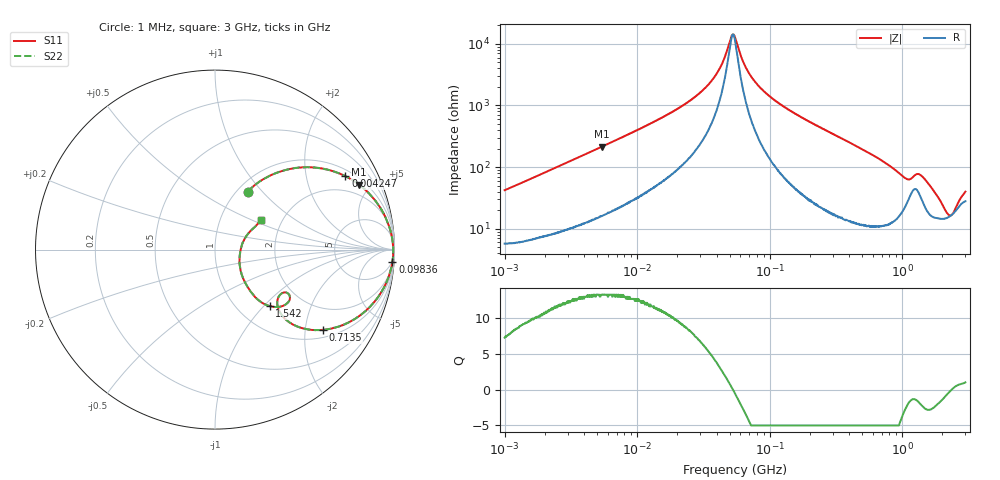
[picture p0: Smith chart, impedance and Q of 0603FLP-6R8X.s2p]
!s-Parameter Generated by FASTRON Sdn. Bhd.
!FASTRON P/N : 0603FLP-6R8X
!Keysight Technologies: E4991B_MY54100416_A.01.15
!Date: Tue Dec 02 13:07:44 2025
!Version  :Rev00  Tue Dec 02 13:07:44 2025
!Data & Calibration Information:
!Freq  S11  S21  S12  S22
!PortZ  Port1:50+j0  Port2:50+j0
!When reading reference impedance value at option line is always used.
! Remarks : This data is being provided solely for informational purposes.
# Hz S dB R 50
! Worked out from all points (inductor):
!   1601 points, 1 MHz to 3 GHz, reference 50 ohm
!   read as one part in series: L = 6.55 uH near 1.041 MHz
!   highest Q = 13.3 at 5.4 MHz (marker M1), where L = 6.29 uH
!   self-resonance near 52.62 MHz
!   S11 on the Smith chart (normalised r, x): 1 MHz: 1.11, +0.84; 4.247 MHz: 1.26, +3.38; 98.36 MHz: 4, -29; 713.5 MHz: 1.22, -2.50; 1.542 GHz: 1.39, -1.08; 3 GHz: 1.56, +0.57
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1000000  -8.60 60.6  -1.12 -21.6  -1.12 -21.6  -8.60 60.6
2128890  -4.06 46.2  -2.80 -38.6  -2.80 -38.6  -4.06 46.2
3804036  -1.86 32.0  -5.49 -53.6  -5.49 -53.6  -1.86 32.0
4246734  -1.58 29.4  -6.14 -56.2  -6.14 -56.2  -1.58 29.4
5399688  -1.10 24.2  -7.71 -61.5  -7.71 -61.5  -1.10 24.2
1.447069e7  -0.25 9.4  -15.70 -75.5  -15.70 -75.5  -0.25 9.4
3.371011e7  -0.08 2.7  -26.40 -77.2  -26.40 -77.2  -0.08 2.7
4.243531e7  -0.07 1.3  -32.50 -70.2  -32.50 -70.2  -0.07 1.3
5.15801e7  -0.06 0.1  -42.60 -19.8  -42.60 -19.8  -0.06 0.1
5.504702e7  -0.06 -0.2  -41.90 30.5  -41.90 30.5  -0.06 -0.2
6.929487e7  -0.06 -1.6  -30.80 75.2  -30.80 75.2  -0.06 -1.6
9.836149e7  -0.08 -3.9  -23.30 80.4  -23.30 80.4  -0.08 -3.9
2.083556e8  -0.24 -10.8  -14.60 76.2  -14.60 76.2  -0.24 -10.8
4.135554e8  -0.84 -22.0  -8.53 65.0  -8.53 65.0  -0.84 -22.0
7.135306e8  -2.50 -36.6  -4.46 48.3  -4.46 48.3  -2.50 -36.6
7.925923e8  -3.15 -40.0  -3.79 43.8  -3.79 43.8  -3.15 -40.0
1.033307e9  -6.06 -43.8  -2.76 28.3  -2.76 28.3  -6.06 -43.8
1.194682e9  -6.94 -32.2  -3.55 21.2  -3.55 21.2  -6.94 -32.2
1.333714e9  -5.99 -34.4  -3.73 25.8  -3.73 25.8  -5.99 -34.4
1.542004e9  -7.16 -45.9  -2.35 24.4  -2.35 24.4  -7.16 -45.9
2.278218e9  -17.00 -13.2  -1.28 2.1  -1.28 2.1  -17.00 -13.2
3e9  -10.30 33.0  -2.35 -12.6  -2.35 -12.6  -10.30 33.0
